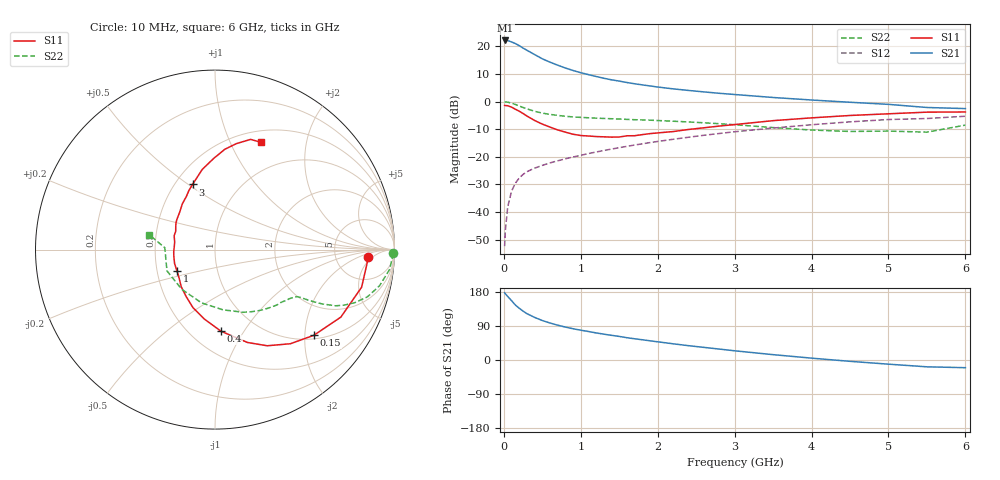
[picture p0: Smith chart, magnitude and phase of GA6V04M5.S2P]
! Infineon Technologies  Discrete & RF Semiconductors
! BF775
! Si NPN RF Bipolar Junction Transistor in SOT23
! VCE = 6 V  IC = 4.5 mA
! Common Emitter S-Parameters:  May  1996
# GHz  S  MA  R  50
!  f  S11  S21  S12  S22
! GHz  MAG  ANG  MAG  ANG  MAG  ANG  MAG  ANG
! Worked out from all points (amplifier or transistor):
!   36 points, 10 MHz to 6 GHz, reference 50 ohm
!   highest |S21| = 22.2 dB at 20 MHz (marker M1)
!   |S21| within 3 dB of that: start of sweep to 264.8 MHz
!   unconditionally stable (mu >= 1): 864.6 MHz to 3.152 GHz
!   at 250 MHz: K = 0.45, MSG = 22.9 dB, |S12| = -26.4 dB
!   at 1.4 GHz: K = 1.11, MAG = 10.5 dB, |S12| = -17.2 dB
!   at 6 GHz: K = 0.92, MSG = 1.4 dB, |S12| = -5.3 dB
!   S11 on the Smith chart (normalised r, x): 10 MHz: 12, -4; 150 MHz: 1.09, -2.22; 400 MHz: 0.69, -0.80; 1 GHz: 0.64, -0.16; 3 GHz: 0.61, +0.52; 6 GHz: 0.63, +1.31
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0.01  0.8558 -2.9  12.8 177.5  0.0024 90.2  0.9945 -1.2
0.02  0.8497 -5.7  12.86 174.7  0.0047 82.5  0.9892 -2.6
0.05  0.8433 -14.4  12.8 167.7  0.0123 80.9  0.9789 -6.5
0.1  0.7957 -28.2  12.09 156.6  0.0238 75.0  0.9386 -12.4
0.15  0.729 -40.9  11.31 145.1  0.0333 69.2  0.8893 -17.2
0.2  0.672 -51.3  10.36 136.6  0.0413 65.4  0.8346 -20.7
0.25  0.6097 -61.5  9.355 129.0  0.048 61.4  0.7849 -23.2
0.3  0.5484 -70.7  8.541 122.3  0.0537 59.5  0.741 -25.0
0.4  0.4559 -85.8  7.14 112.4  0.0623 57.2  0.6687 -26.9
0.5  0.3919 -98.6  5.981 104.2  0.0699 56.2  0.6196 -27.9
0.6  0.3457 -110.8  5.195 97.6  0.0776 56.0  0.5879 -28.5
0.8  0.2799 -132.2  4.073 86.9  0.0921 56.3  0.5436 -29.3
1  0.2432 -150.3  3.348 78.7  0.1065 57.3  0.5186 -30.6
1.1  0.2382 -160.9  3.089 75.2  0.1146 57.6  0.5103 -31.6
1.3  0.2304 -176.6  2.655 68.2  0.1302 57.8  0.4957 -33.6
1.6  0.2404 161.2  2.221 58.8  0.1548 57.5  0.4768 -37.4
2.2  0.2869 133.2  1.706 42.8  0.2079 55.0  0.4422 -47.3
3  0.3841 109.0  1.348 24.3  0.2845 48.6  0.3821 -66.0
3.5  0.4526 99.0  1.19 14.1  0.3322 43.3  0.3386 -82.4
4.5  0.5616 84.4  0.975 -3.5  0.4306 31.0  0.2884 -129.9
5.5  0.6453 72.1  0.784 -18.0  0.4948 15.8  0.2799 177.9
6  0.65 66.9  0.749 -20.3  0.5442 11.5  0.3759 167.2
